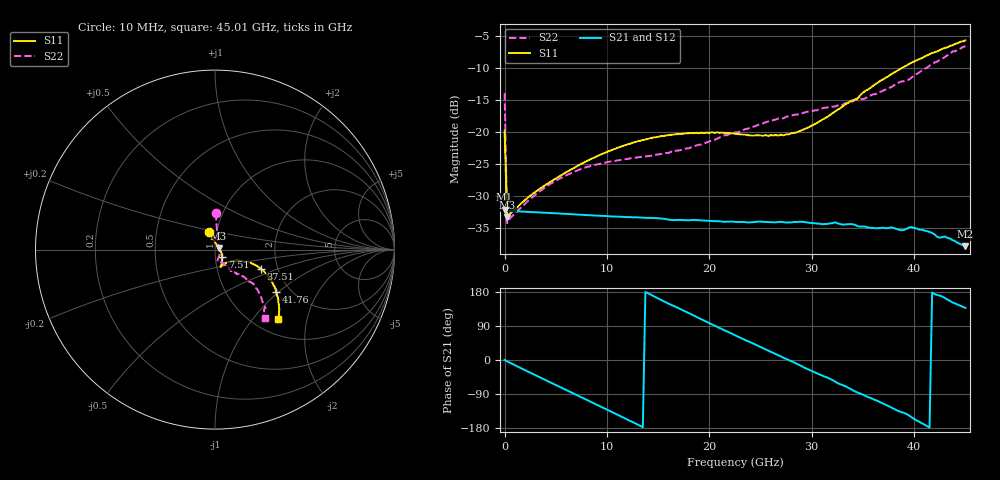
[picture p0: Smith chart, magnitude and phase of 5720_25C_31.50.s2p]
! Device:  ADRF5720
! Description: 0.5dB LSB GaAs MMIC 6-bit Digital Attenuator
! Frequency:  0.000009 -  40 GHz
! Ports:
!	RF1	= Port 1
!	RF2	= Port 2
! Vdd:  3.3 Volt
! Vss:  -3.3 Volt
! Control:  0/3.3 Volt
! State:  31.50 dB attenuation
! Data:  The device was measured using G-S-G Probes on a matrix board.
!  Data was collected using an calibrated 4 port network analyzer.
!  The reference plane for this measurement is at the launchers.
! Note:  Analog Devices supplies this data as a sample of measured data
!  for this product.  Your particular data for this product may vary.
!  Data was taken at 25 degrees C.
!  Analog Devices reserves the right to change this data at anytime.
# GHZ S DB R 45.0
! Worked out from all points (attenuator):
!   181 points, 10 MHz to 45.01 GHz, reference 45 ohm
!   highest |S21| = -32.05 dB at 10 MHz (marker M1); lowest = -37.8 dB at 45.01 GHz (marker M2)
!   lowest |S11| = -33.2 dB at 260 MHz (marker M3), VSWR 1.04, Z = 46.8 + j0.875 ohm
!   |S11| at or under -10 dB: start of sweep to 38.74 GHz
!   |S22| runs from -34.2 to -6.5 dB; largest |S21 - S12| = 0.00013
!   S11 on the Smith chart (normalised r, x): 10 MHz: 0.92, +0.18; 7.51 GHz: 1.08, -0.09; 37.51 GHz: 1.63, -0.37; 41.76 GHz: 1.69, -0.97; 45.01 GHz: 1.27, -1.35
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0.01  -19.73 109.2  -32.05 0.2  -32.06 0.3  -13.86 88.8
0.26  -33.24 25.4  -32.24 -3.6  -32.24 -3.7  -34.17 25.1
0.51  -32.73 14.0  -32.26 -7.0  -32.27 -7.0  -33.43 10.8
3.26  -29.00 -18.9  -32.48 -43.3  -32.47 -43.3  -29.39 -38.0
5.01  -27.19 -32.9  -32.63 -66.0  -32.62 -66.0  -27.51 -55.3
7.51  -24.89 -46.2  -32.85 -98.4  -32.85 -98.4  -25.71 -68.8
7.76  -24.68 -47.3  -32.88 -101.7  -32.87 -101.7  -25.55 -70.0
11.51  -22.13 -59.8  -33.19 -150.7  -33.19 -150.6  -24.21 -76.2
15.26  -20.59 -67.6  -33.44 158.9  -33.44 158.9  -23.36 -72.4
20.26  -19.97 -71.3  -33.83 93.7  -33.83 93.7  -21.27 -60.2
22.76  -20.26 -69.3  -33.98 62.2  -33.98 62.2  -19.98 -56.3
27.26  -20.47 -51.6  -34.01 5.6  -34.01 5.6  -17.78 -53.3
30.26  -18.75 -33.5  -34.17 -31.9  -34.17 -31.9  -16.56 -52.9
32.26  -16.74 -25.3  -34.05 -56.4  -34.05 -56.2  -15.95 -51.0
34.51  -14.67 -20.7  -34.65 -86.1  -34.64 -86.0  -14.93 -48.6
35.01  -13.79 -20.2  -34.68 -91.3  -34.68 -91.2  -14.81 -47.9
37.51  -11.20 -22.6  -34.92 -121.4  -34.94 -121.3  -13.05 -43.4
37.76  -10.91 -23.2  -34.82 -125.1  -34.87 -124.9  -12.95 -43.2
38.76  -9.98 -25.2  -35.27 -137.6  -35.22 -137.6  -12.05 -43.5
39.76  -9.10 -28.5  -34.77 -151.2  -34.80 -150.9  -11.42 -42.3
41.76  -7.61 -34.8  -35.69 177.8  -35.65 177.7  -9.37 -44.2
45.01  -5.64 -47.9  -37.76 137.6  -37.76 138.0  -6.53 -54.0
